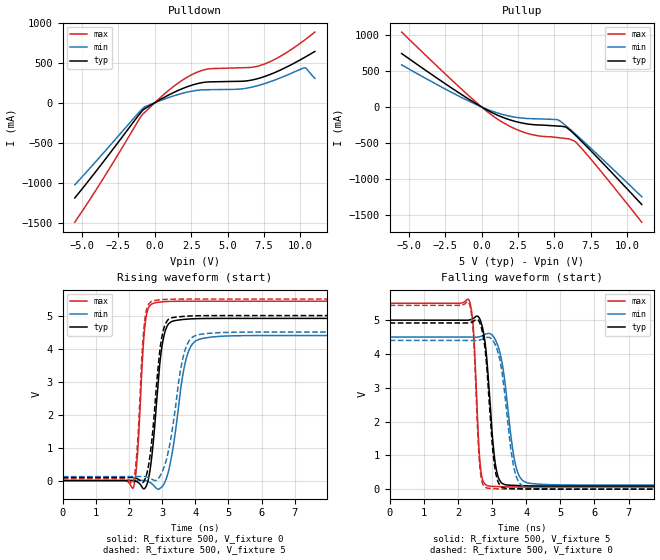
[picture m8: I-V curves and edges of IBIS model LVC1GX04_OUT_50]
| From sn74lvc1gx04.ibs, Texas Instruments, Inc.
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[Model]   LVC1GX04_OUT_50
Model_type  Output
Vref =   0
Rref =   500
Cref =   50p
Vmeas =   2.5
| variable   typ   min   max
C_comp   8.96pF   5.46pF   12.43pF
| C_pullup   9.71pF   5.46pF   12.43pF
| C_pulldown   8.21pF   6.24pF   11.46pF
[Temperature Range]   40   100   -40
| Ambient temperature   25   85   -40
[Voltage range]   5   4.5   5.5
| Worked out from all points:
|   slope of the pulldown table from 0 to 0.75 V, typ, clamps not added: 9.73 ohm
|   slope of the pullup table from 0 to 0.75 V, typ, clamps not added: 9.16 ohm
|   rising waveform, R_fixture 500, V_fixture 0: 20-80 % time 261ps typ, 374ps min, 173ps max; typ from 0 V to 4.91 V
|   falling waveform, R_fixture 500, V_fixture 5: 20-80 % time 226ps typ, 321ps min, 148ps max; typ from 5 V to 0.091 V
|   rising waveform, R_fixture 500, V_fixture 5: 20-80 % time 267ps typ, 397ps min, 175ps max; typ from 0.091 V to 5 V
|   falling waveform, R_fixture 500, V_fixture 0: 20-80 % time 222ps typ, 314ps min, 144ps max; typ from 4.92 V to 0 V
[Pulldown]
| LVC1GX04_OUT_50
|   Voltage   I(typ)   I(min)   I(max)
-5.5V     -1.19A     -1.026A    -1.493A
-3.615V   -756.5mA   -644.9mA   -968mA
-860mV    -99.61mA   -76.72mA   -149.6mA
1.145V    114mA      76.72mA    182.7mA
2.335V    206.5mA    136.8mA    330.4mA
3.39V     254.8mA    162mA      411mA
5.9V      268mA      171.6mA    436.9mA
6.79V     288.1mA    200.2mA    446mA
7.59V     330.6mA    241.7mA    487.6mA
8.82V     424.5mA    324.7mA    600.5mA
10.29V    565.4mA    436.9mA    781.9mA
11V       641.1mA    304.6mA    882.6mA
[Pullup]
| LVC1GX04_OUT_50
|   Voltage   I(typ)   I(min)   I(max)
-5.5V     745.2mA    587.5mA    1.044A
-1.18V    147.6mA    112.6mA    211.7mA
1.04V     -109.2mA   -79.97mA   -161.6mA
2.045V    -185.4mA   -131.8mA   -280mA
3.05V     -232.7mA   -158.7mA   -361.3mA
3.945V    -250.5mA   -165.3mA   -402.5mA
5.295V    -265.8mA   -184.8mA   -427.6mA
5.83V     -285.1mA   -267.5mA   -440mA
6.335V    -372.8mA   -357.2mA   -470.5mA
6.54V     -412.8mA   -394.7mA   -503.8mA
8.12V     -739mA     -692.4mA   -876.8mA
11V       -1.358A    -1.25A     -1.605A
[Ramp]
| LVC1GX04_OUT_50
| variable   typ   min   max
dV/dt_r   3.10/2.87E-10   2.79/4.03E-10   3.40/1.85E-10
dV/dt_f   3.02/2.39E-10   2.69/3.36E-10   3.34/1.55E-10
R_load = 500
[Rising Waveform]
| LVC1GX04_OUT_50
R_fixture =   500
C_fixture =   0
L_fixture =   0
V_fixture =   0
V_fixture_min = 0
V_fixture_max = 0
|   Time   V(typ)   V(min)   V(max)
0s        185.3pV    4.77nV     2.097nV
2.13ns    -827.3uV   290.3uV    -217.4mV
2.25ns    -42.01mV   1.447mV    722.8mV
2.485ns   -223.8mV   -1.585mV   4.742V
2.78ns    1.718V     -190.1mV   5.386V
2.96ns    3.825V     -218.6mV   5.412V
3.145ns   4.669V     120.6mV    5.425V
3.72ns    4.89V      3.675V     5.435V
4.23ns    4.91V      4.31V      5.435V
24.99ns   4.914V     4.397V     5.435V
[Falling Waveform]
| LVC1GX04_OUT_50
R_fixture =   500
C_fixture =   0
L_fixture =   0
V_fixture =   5
V_fixture_min = 4.5
V_fixture_max = 5.5
|   Time   V(typ)   V(min)   V(max)
0s        5V         4.5V       5.5V
2.325ns   5.004V     4.499V     5.595V
2.455ns   5.053V     4.497V     4.729V
2.655ns   5.004V     4.515V     717.4mV
2.87ns    3.567V     4.604V     103mV
3.045ns   1.198V     4.509V     80.99mV
3.185ns   344.2mV    4.199V     74.93mV
3.685ns   110.3mV    735.9mV    65.22mV
4.085ns   97.75mV    175.5mV    63.6mV
24.99ns   91.35mV    120.7mV    62.83mV
[Rising Waveform]
| LVC1GX04_OUT_50
R_fixture =   500
C_fixture =   0
L_fixture =   0
V_fixture =   5
V_fixture_min = 4.5
V_fixture_max = 5.5
|   Time   V(typ)   V(min)   V(max)
0s        91.33mV    120.7mV    62.82mV
2.11ns    93.26mV    120.9mV    -82.38mV
2.24ns    59.96mV    122mV      904.3mV
2.475ns   30.41mV    121mV      4.863V
2.77ns    2.132V     4.648mV    5.455V
2.93ns    3.949V     131.5mV    5.476V
3.1ns     4.754V     537.9mV    5.489V
3.655ns   4.976V     3.832V     5.499V
4.13ns    4.996V     4.428V     5.5V
24.99ns   5V         4.5V       5.5V
[Falling Waveform]
| LVC1GX04_OUT_50
R_fixture =   500
C_fixture =   0
L_fixture =   0
V_fixture =   0
V_fixture_min = 0
V_fixture_max = 0
|   Time   V(typ)   V(min)   V(max)
0s        4.917V     4.401V     5.437V
2.32ns    4.92V      4.4V       5.523V
2.45ns    4.964V     4.398V     4.648V
2.645ns   4.914V     4.413V     648.4mV
2.865ns   3.361V     4.492V     32.05mV
3.025ns   1.136V     4.399V     16.39mV
3.17ns    238.6mV    4.061V     10.65mV
3.645ns   15.65mV    622.3mV    2.33mV
4.01ns    6.104mV    50.58mV    850.8uV
24.99ns   16.36uV    24.58uV    11.82uV
